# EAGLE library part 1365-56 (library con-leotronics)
DUAL ROW STRAIGHT HEADER 1364 SERIES. 1.27mm x 1.27mm. Without Fixing Post. SMT Source: http://www.leotronics.co.uk/Conexcon/Data%20Sheets/sec.%20A/1364ing.pdf
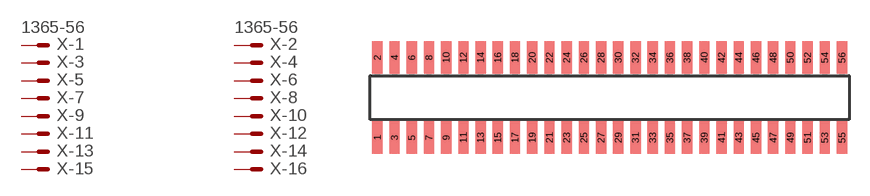
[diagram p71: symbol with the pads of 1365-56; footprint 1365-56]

Designator prefix X; gates -1=MVAL -2=MVAL -3=M -4=M -5=M -6=M -7=M -8=M -9=M -10=M -11=M -12=M -13=M -14=M -15=M -16=M -17=M -18=M -19=M -20=M -21=M -22=M -23=M -24=M -25=M -26=M -27=M -28=M -29=M -30=M -31=M -32=M -33=M -34=M -35=M -36=M -37=M -38=M -39=M -40=M -41=M -42=M -43=M -44=M -45=M -46=M -47=M -48=M -49=M -50=M -51=M -52=M -53=M -54=M -55=M -56=M

## 1365-56 (OC_FARNELL: unknown; OC_NEWARK: unknown)  [1365-56]
1  -1:S  pas
2  -2:S  pas
3  -3:S  pas
4  -4:S  pas
5  -5:S  pas
6  -6:S  pas
7  -7:S  pas
8  -8:S  pas
9  -9:S  pas
10  -10:S  pas
11  -11:S  pas
12  -12:S  pas
13  -13:S  pas
14  -14:S  pas
15  -15:S  pas
16  -16:S  pas
17  -17:S  pas
18  -18:S  pas
19  -19:S  pas
20  -20:S  pas
21  -21:S  pas
22  -22:S  pas
23  -23:S  pas
24  -24:S  pas
25  -25:S  pas
26  -26:S  pas
27  -27:S  pas
28  -28:S  pas
29  -29:S  pas
30  -30:S  pas
31  -31:S  pas
32  -32:S  pas
33  -33:S  pas
34  -34:S  pas
35  -35:S  pas
36  -36:S  pas
37  -37:S  pas
38  -38:S  pas
39  -39:S  pas
40  -40:S  pas
41  -41:S  pas
42  -42:S  pas
43  -43:S  pas
44  -44:S  pas
45  -45:S  pas
46  -46:S  pas
47  -47:S  pas
48  -48:S  pas
49  -49:S  pas
50  -50:S  pas
51  -51:S  pas
52  -52:S  pas
53  -53:S  pas
54  -54:S  pas
55  -55:S  pas
56  -56:S  pas

## Footprint 1365-56 (pad centres in mm)
DUAL ROW STRAIGHT HEADER 1364 SERIES. 1.27mm x 1.27mm. Without Fixing Post. SMT Source: http://www.leotronics.co.uk/Conexcon/Data%20Sheets/sec.%20A/1364ing.pdf
smd 0.76 x 2.4: 1 -17.145,-2.95; 2 -17.145,2.95; 3 -15.875,-2.95; 4 -15.875,2.95; 5 -14.605,-2.95; 6 -14.605,2.95; 7 -13.335,-2.95; 8 -13.335,2.95; 9 -12.065,-2.95; 10 -12.065,2.95; 11 -10.795,-2.95; 12 -10.795,2.95; 13 -9.525,-2.95; 14 -9.525,2.95; 15 -8.255,-2.95; 16 -8.255,2.95; 17 -6.985,-2.95; 18 -6.985,2.95; 19 -5.715,-2.95; 20 -5.715,2.95; 21 -4.445,-2.95; 22 -4.445,2.95; 23 -3.175,-2.95; 24 -3.175,2.95; 25 -1.905,-2.95; 26 -1.905,2.95; 27 -0.635,-2.95; 28 -0.635,2.95; 29 0.635,-2.95; 30 0.635,2.95; 31 1.905,-2.95; 32 1.905,2.95; 33 3.175,-2.95; 34 3.175,2.95; 35 4.445,-2.95; 36 4.445,2.95; 37 5.715,-2.95; 38 5.715,2.95; 39 6.985,-2.95; 40 6.985,2.95; 41 8.255,-2.95; 42 8.255,2.95; 43 9.525,-2.95; 44 9.525,2.95; 45 10.795,-2.95; 46 10.795,2.95; 47 12.065,-2.95; 48 12.065,2.95; 49 13.335,-2.95; 50 13.335,2.95; 51 14.605,-2.95; 52 14.605,2.95; 53 15.875,-2.95; 54 15.875,2.95; 55 17.145,-2.95; 56 17.145,2.95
